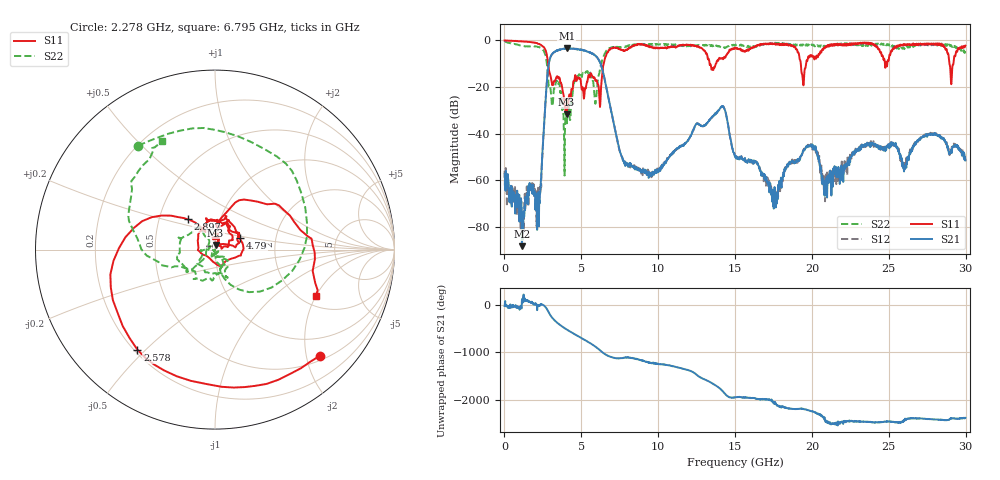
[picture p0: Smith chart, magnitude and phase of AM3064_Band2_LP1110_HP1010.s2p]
# Hz S DB R 50.0
!freq dBS11 angS11 dBS21 angS21 dBS12 angS12 dBS22 angS22
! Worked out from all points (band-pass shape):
!   1600 points, 10 MHz to 29.98 GHz, reference 50 ohm
!   highest |S21| = -3.36 dB at 4.059 GHz (marker M1); lowest = -88.2 dB at 1.135 GHz (marker M2)
!   |S21| within 3 dB of the highest: 3.05 GHz to 5.882 GHz (2.832 GHz wide, 63.4 % of centre)
!   lowest |S11| = -31.7 dB at 4.04 GHz (marker M3), VSWR 1.05, Z = 50.3 + j2.59 ohm
!   |S11| at or under -10 dB: 2.837 GHz to 6.451 GHz (3.614 GHz wide, 77.8 % of centre); 13.34 GHz to 13.75 GHz (406.3 MHz wide, 3 % of centre); 19.27 GHz to 19.62 GHz (340.8 MHz wide, 1.75 % of centre)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
!   |S22| runs from -57.9 to -0.2 dB; largest |S21 - S12| = 0.022
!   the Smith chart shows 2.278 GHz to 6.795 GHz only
!   S11 on the Smith chart (normalised r, x): 2.278 GHz: 0.59, -2.27; 2.578 GHz: 0.21, -0.47; 2.897 GHz: 0.70, +0.25; 4.79 GHz: 1.31, +0.17; 6.795 GHz: 2.38, -1.99
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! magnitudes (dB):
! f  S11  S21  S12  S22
! 10 MHz  0.0  -57.2  -55.9  -0.2
! 1.135 GHz  -0.4  -88.2  -79.5  -2.3
! 2.278 GHz  -1.6  -69.9  -67.6  -2.9
! 2.578 GHz  -3.0  -36.1  -36.1  -4.8
! 2.897 GHz  -12.8  -9.5  -9.4  -19.7
! 4.04 GHz  -31.7  -3.6  -3.3  -33.4
! 4.059 GHz  -30.6  -3.4  -3.5  -35.6
! 4.79 GHz  -16.3  -3.8  -3.7  -15.8
! 5.015 GHz  -20.4  -4.1  -4.0  -15.3
! 5.933 GHz  -17.3  -6.6  -6.6  -26.6
! 6.795 GHz  -4.2  -25.6  -25.6  -3.4
! 7.826 GHz  -4.4  -52.5  -52.9  -2.8
! 10 GHz  -3.4  -55.4  -55.8  -1.8
! 14.14 GHz  -7.6  -28.4  -28.4  -3.0
! 15 GHz  -3.3  -49.8  -49.4  -1.9
! 17.63 GHz  -1.7  -65.0  -65.2  -1.1
! 19.99 GHz  -6.4  -45.2  -45.1  -1.7
! 20.85 GHz  -3.1  -66.5  -69.0  -2.4
! 25 GHz  -8.4  -45.4  -44.6  -1.7
! 28.28 GHz  -1.3  -41.1  -40.9  -2.5
! 29.08 GHz  -17.5  -46.6  -46.5  -2.5
! 29.98 GHz  -2.3  -51.4  -51.6  -4.5
